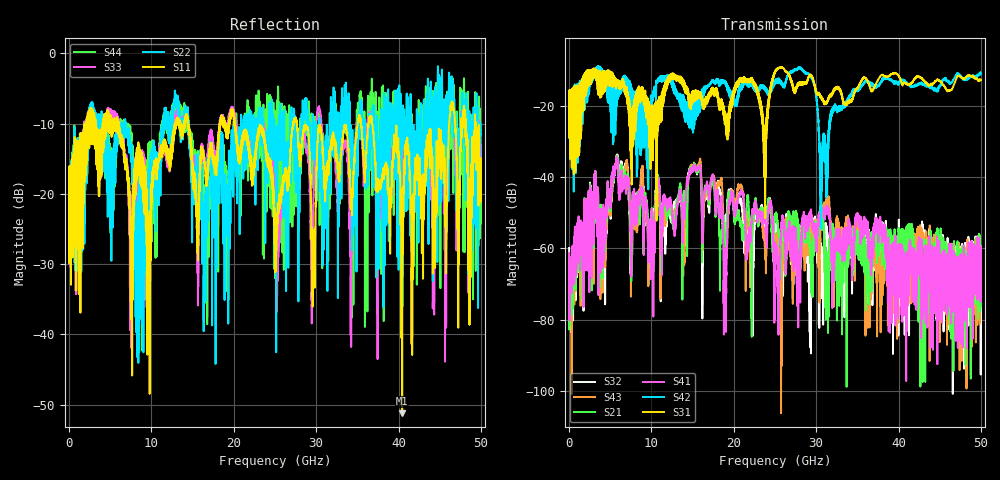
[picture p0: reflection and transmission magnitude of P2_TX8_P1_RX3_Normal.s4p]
!Keysight Technologies,N5225B,MY57041031,A.13.20.10
!Date: Friday, May 31, 2019 11:18:40
!Correction: S11(Full 4 Port(1,2,3,4))
!S12(Full 4 Port(1,2,3,4))
!S13(Full 4 Port(1,2,3,4))
!S14(Full 4 Port(1,2,3,4))
!S21(Full 4 Port(1,2,3,4))
!S22(Full 4 Port(1,2,3,4))
!S23(Full 4 Port(1,2,3,4))
!S24(Full 4 Port(1,2,3,4))
!S31(Full 4 Port(1,2,3,4))
!S32(Full 4 Port(1,2,3,4))
!S33(Full 4 Port(1,2,3,4))
!S34(Full 4 Port(1,2,3,4))
!S41(Full 4 Port(1,2,3,4))
!S42(Full 4 Port(1,2,3,4))
!S43(Full 4 Port(1,2,3,4))
!S44(Full 4 Port(1,2,3,4))
!S4P File: Measurements: <S11,S12,S13,S14>,
!<S21,S22,S23,S24>,
!<S31,S32,S33,S34>,
!<S41,S42,S43,S44>:
# Hz S  dB  R 50.0
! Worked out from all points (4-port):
!   5000 points, 10 MHz to 50 GHz, reference 50 ohm
!   strongest paths, dB at 10 MHz, 12.51 GHz, 25.01 GHz, 37.51 GHz, 50 GHz:
!     S31: -19.3, -11.5, -10.3, -12.8, -12.8
!     S42: -19.7, -14.5, -13.0, -14.3, -11.1
!     S41: -61.4, -50.1, -68.0, -53.4, -68.4
!     S21: -66.2, -51.6, -51.5, -56.6, -63.3
!     S43: -63.5, -50.9, -62.7, -61.5, -71.7
!     S32: -59.9, -51.8, -55.7, -58.5, -66.6
!   lowest |S11| = -51.2 dB at 40.44 GHz (marker M1), VSWR 1.01, Z = 50 - j0.272 ohm
!   |S11| at or under -10 dB: 20.17 GHz to 27.18 GHz (7.014 GHz wide, 29.6 % of centre); 27.67 GHz to 35.04 GHz (7.368 GHz wide, 23.5 % of centre); 36.81 GHz to 46.16 GHz (9.35 GHz wide, 22.5 % of centre)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
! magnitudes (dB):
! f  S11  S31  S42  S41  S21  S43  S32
! 10 MHz  -19.6  -19.3  -19.7  -61.4  -66.2  -63.5  -59.9
! 5.72 GHz  -10.6  -13.6  -22.9  -35.5  -35.3  -35.1  -35.2
! 9.77 GHz  -24.5  -20.3  -29.7  -56.5  -55.0  -59.8  -59.6
! 28.07 GHz  -15.2  -13.4  -9.4  -75.3  -60.4  -56.4  -59.4
! 30.63 GHz  -11.5  -17.5  -40.5  -48.6  -49.5  -51.8  -59.5
! 40.44 GHz  -51.2  -14.2  -12.8  -66.6  -59.2  -56.3  -58.8
! 50 GHz  -15.0  -12.8  -11.1  -68.4  -63.3  -71.7  -66.6
